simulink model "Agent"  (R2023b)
settings: Solver=ode3  StartTime=0.0  StopTime=t_end  FixedStep=dt8dof  RelTol=1e-3
PreLoadFcn:
  | define_swarm_buses(3, 1000);
model workspace (MAT data in the model file):
  dt8dof = 0.002
  dtastar = 0.1
  dtcontrol = 0.03
  id = 1
  phi_road0 = 0
  psi0 = 0
  slope_x_body0 = 0
  slope_y_body0 = 0
  t_end = 70
  teta0 = 0
  tetapunto0 = 0
  theta_road0 = 0
  velstart = 5
  wr0_FL = 3.15
  wr0_FR = 3.15
  wr0_RL = 3.15
  wr0_RR = 3.15
  x0 = 0
  y0 = 0
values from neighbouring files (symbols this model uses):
  scenario = evalin('base', 'scenario')    [apply_map_event.m]    (also in obstacle_brake_from_base.m; swarm_planner_helper2.m)

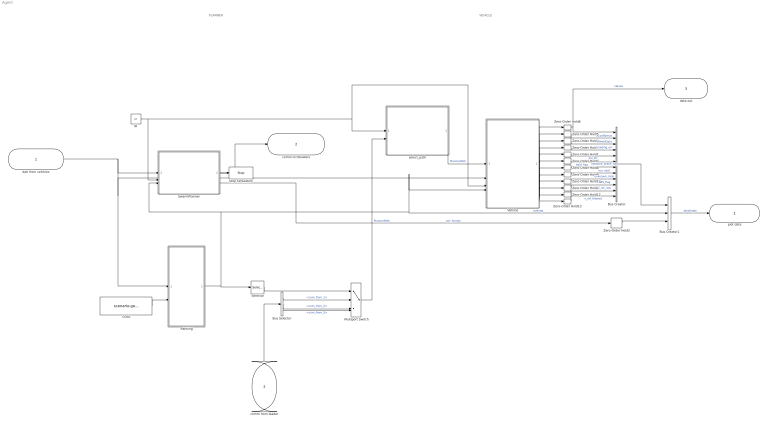
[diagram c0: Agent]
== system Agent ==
  note: PLANNER
  note: VEHICLE
  dati from vehicles : Inport  OutDataTypeStr=Bus: ValuesBus
  comm from leader : Inport  Port=2  OutDataTypeStr=Bus: PlannerOutBusGlobal  SampleTime=dtastar
  Bus Creator : BusCreator  Inputs=12  OutDataTypeStr=Bus: PlotVeicolo
  Bus Creator1 : BusCreator  Inputs=3  OutDataTypeStr=Bus: PlotSingle
  Bus Selector : BusSelector  OutputSignals=com_from_1,com_from_2,com_from_3
  GOAL : Constant  Value=scenario.goal
  ID : Constant  Value=id
  Multiport Switch : MultiPortSwitch
  Ranking : MATLAB Function  TreatAsAtomicUnit=on
  Selector : Selector  InputPortWidth=3  IndexOptions=Index vector (dialog)  Indices=[1]  OutputSizes=1
  Stop Simulation : Stop
  SwarmPlanner : MATLAB Function  TreatAsAtomicUnit=on
  Vehicle : ModelReference  ModelNameDialog=vehicle  UsingDefaultArgumentValue=0,0,0,0,0,0,0,0,0,0,0,0,0,0  SimulationMode=Normal  ModelReferenceVersion=1.119
  Zero-Order Hold{1..13} (13 alike) : ZeroOrderHold  SampleTime=dtastar
  select_path : MATLAB Function  TreatAsAtomicUnit=on
  plot data : Outport  OutDataTypeStr=Bus: PlotSingle  SampleTime=dtastar
  comm to followers : Outport  Port=2  OutDataTypeStr=Bus: PlannerOutBusSingle
  data out : Outport  Port=3  OutDataTypeStr=Bus: VehicleState
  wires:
  comm from leader/1 -> Bus Selector/1
  SwarmPlanner/1(PlannerOutBusSingle) -> comm to followers/1
  Bus Creator1/1 -> plot data/1  "plotsingle"
  ID/1 -> Vehicle/3, select_path/1(id), SwarmPlanner/2(id)
  Ranking/1(ranking) -> Selector/1, SwarmPlanner/3(ranking), Vehicle/4, Bus Creator1/2  "ranking"
  GOAL/1 -> Ranking/2(goal)
  Vehicle/2 -> Zero-Order Hold5/1
  Multiport Switch/1 -> select_path/2(Bus)  "PlannerPath"
  dati from vehicles/1 -> Ranking/1(ValuesBus), Vehicle/2, SwarmPlanner/1(ValuesBus)
  Vehicle/1 -> Zero-Order Hold6/1
  Bus Selector/1 -> Multiport Switch/2  "<com_from_1>"
  Bus Selector/2 -> Multiport Switch/3  "<com_from_2>"
  Bus Selector/3 -> Multiport Switch/4  "<com_from_3>"
  select_path/1(my_planner_data) -> Vehicle/1  "PlannerPath"
  SwarmPlanner/3(pct_known) -> Zero-Order Hold2/1  "pct_known"
  Bus Creator/1 -> Bus Creator1/1
  Vehicle/3 -> Zero-Order Hold4/1
  SwarmPlanner/2(goal_flag) -> Stop Simulation/1
  Zero-Order Hold2/1 -> Bus Creator1/3
  Selector/1 -> Multiport Switch/1
  Vehicle/5 -> Zero-Order Hold1/1
  Vehicle/4 -> Zero-Order Hold3/1
  Zero-Order Hold1/1 -> Bus Creator/5  "psi_err"
  Zero-Order Hold3/1 -> Bus Creator/4  "heading_err"
  Zero-Order Hold4/1 -> Bus Creator/3  "WheelData"
  Zero-Order Hold5/1 -> Bus Creator/2  "AccelSterzo"
  Zero-Order Hold6/1 -> Bus Creator/1, data out/1  "values"
  Zero-Order Hold7/1 -> Bus Creator/6  "obstacle_brake_flag"
  Vehicle/6 -> Zero-Order Hold7/1
  Zero-Order Hold8/1 -> Bus Creator/7  "hold_flag"
  Vehicle/7 -> Zero-Order Hold8/1
  Vehicle/8 -> Zero-Order Hold9/1
  Vehicle/12 -> Zero-Order Hold13/1
  Vehicle/11 -> Zero-Order Hold12/1
  Vehicle/10 -> Zero-Order Hold11/1
  Vehicle/9 -> Zero-Order Hold10/1
  Zero-Order Hold9/1 -> Bus Creator/8  "mu_next"
  Zero-Order Hold10/1 -> Bus Creator/9  "unknown_ratio"
  Zero-Order Hold11/1 -> Bus Creator/10  "ABS_flag"
  Zero-Order Hold12/1 -> Bus Creator/11  "v_ref_raw"
  Zero-Order Hold13/1 -> Bus Creator/12  "v_ref_filtered"
  ? -> ?

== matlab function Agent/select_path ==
function my_planner_data = select_my_path(id, Bus)
%SELECT_MY_PATH Estrae il PlannerPath del veicolo corrente.
%#codegen

my_planner_data = Bus.id1;

switch int32(id)
    case 1
        my_planner_data = Bus.id1;

    case 2
        my_planner_data = Bus.id2;

    case 3
        my_planner_data = Bus.id3;

    otherwise
        my_planner_data = Bus.id1;
end

end

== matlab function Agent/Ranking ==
function ranking = classifica(ValuesBus, goal)
%CLASSIFICA Ranking decentralizzato pesato:
% 70% distanza dal goal + 30% ETA radiale al goal, con isteresi.
%
% Score basso = veicolo migliore.
%
%#codegen

%% Parametri
N_VEH = 3;

W_DIST = 0.70;
W_ETA  = 0.30;

HYST_FRAC = 0.20;

% Velocita' radiale minima utile verso il goal.
% Sotto questa soglia considero l'ETA non affidabile.
V_RAD_EPS = 0.20;     % [m/s]

% Valore normalizzato assegnato a veicoli che non stanno andando verso il goal.
% 2.0 = penalita' moderata, non infinita.
% Se vuoi punire di piu' chi va nella direzione sbagliata, metti 3.0.
ETA_BAD_NORM = 2.0;

DIST_EPS = 1e-6;
ETA_EPS  = 1e-6;

%% Allocazione statica
ids = zeros(N_VEH, 1);

xs  = zeros(N_VEH, 1);
ys  = zeros(N_VEH, 1);
ps  = zeros(N_VEH, 1);
vs  = zeros(N_VEH, 1);

dist_arr = zeros(N_VEH, 1);
eta_arr  = zeros(N_VEH, 1);
eta_valid = false(N_VEH, 1);

scores = zeros(N_VEH, 1);

%% Raccolta stati statica dal bus

ids(1) = 1;
xs(1)  = ValuesBus.id1.x;
ys(1)  = ValuesBus.id1.y;
ps(1)  = ValuesBus.id1.psi;
vs(1)  = ValuesBus.id1.vel_totale;

ids(2) = 2;
xs(2)  = ValuesBus.id2.x;
ys(2)  = ValuesBus.id2.y;
ps(2)  = ValuesBus.id2.psi;
vs(2)  = ValuesBus.id2.vel_totale;

ids(3) = 3;
xs(3)  = ValuesBus.id3.x;
ys(3)  = ValuesBus.id3.y;
ps(3)  = ValuesBus.id3.psi;
vs(3)  = ValuesBus.id3.vel_totale;

%% Goal
gx = goal(1);
gy = goal(2);

%% Prima passata: calcolo distanze ed ETA radiali
for k = 1:N_VEH

    dx = gx - xs(k);
    dy = gy - ys(k);

    d = sqrt(dx*dx + dy*dy);
    dist_arr(k) = d;

    if d < 1e-3
        eta_arr(k) = 0.0;
        eta_valid(k) = true;
    else
        ux = dx / d;
        uy = dy / d;

        vx = vs(k) * cos(ps(k));
        vy = vs(k) * sin(ps(k));

        % Velocita' proiettata lungo la direzione veicolo -> goal
        v_rad = vx*ux + vy*uy;

        if v_rad > V_RAD_EPS
            eta_arr(k) = d / v_rad;
            eta_valid(k) = true;
        else
            % Veicolo fermo, laterale o che si sta allontanando dal goal.
            eta_arr(k) = 0.0;
            eta_valid(k) = false;
        end
    end
end

%% Normalizzazione distanza
d_ref = max(dist_arr);

if d_ref < DIST_EPS
    d_ref = 1.0;
end

%% Normalizzazione ETA solo sui veicoli validi
eta_ref = 0.0;

for k = 1:N_VEH
    if eta_valid(k)
        if eta_arr(k) > eta_ref
            eta_ref = eta_arr(k);
        end
    end
end

if eta_ref < ETA_EPS
    eta_ref = 1.0;
end

%% Score finale normalizzato
for k = 1:N_VEH

    d_norm = dist_arr(k) / d_ref;

    if eta_valid(k)
        eta_norm = eta_arr(k) / eta_ref;

        % Saturazione: il termine ETA non deve distruggere il peso 70/30.
        if eta_norm > ETA_BAD_NORM
            eta_norm = ETA_BAD_NORM;
        end
    else
        eta_norm = ETA_BAD_NORM;
    end

    scores(k) = W_DIST * d_norm + W_ETA * eta_norm;
end

%% Ordina e applica isteresi
[sorted_sc, idx_sorted] = sort(scores);
new_ranking = ids(idx_sorted);

persistent prev_ranking

if isempty(prev_ranking)
    prev_ranking = new_ranking;
    ranking = new_ranking;
    return;
end

if isequal(new_ranking, prev_ranking)

    ranking = new_ranking;

else

    best_score   = sorted_sc(1);
    second_score = sorted_sc(2);

    % Se il vantaggio del nuovo primo e' piccolo, mantieni il ranking precedente.
    if abs(second_score - best_score) < HYST_FRAC * max(second_score, 1e-6)
        ranking = prev_ranking;
    else
        ranking = new_ranking;
        prev_ranking = new_ranking;
    end

end

end

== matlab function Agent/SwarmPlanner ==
function [PlannerOutBusSingle, goal_flag, pct_known] = ...
    SwarmPlanner(ValuesBus, id, ranking)
%SWARMPLANNER Wrapper Simulink per architettura decentralizzata.
%
% ranking = [id_primo; id_secondo; id_terzo]
%
% path_x_1 = path per il primo classificato
% path_x_2 = path per il secondo classificato
% path_x_3 = path per il terzo classificato
%
% L'output finale viene rimappato su:
% PlannerOutBusSingle.id1 / id2 / id3
%
%#codegen

coder.extrinsic('swarm_planner_rank_to_id');

L        = 1000; 
N_REPLAN = 2;

%% Default scalari
goal_flag = 0.0;
pct_known = 0.0;

%% Default bus output: necessario SEMPRE, anche se non sono leader
z = zeros(L,1);

PlannerOutBusSingle.id1.to_path_tracker.path_x = z;
PlannerOutBusSingle.id1.to_path_tracker.path_y = z;
PlannerOutBusSingle.id1.to_path_tracker.n      = 0.0;
PlannerOutBusSingle.id1.to_speed_governor.mu_next       = 1; %metto mu alta, sarà soltanto la prima del segnale disceto,
% altrimenti lo speederefence governor la prima mu che legge è 0 e porta vref=0
PlannerOutBusSingle.id1.to_speed_governor.unknown_ratio = 0.0;

PlannerOutBusSingle.id2.to_path_tracker.path_x = z;
PlannerOutBusSingle.id2.to_path_tracker.path_y = z;
PlannerOutBusSingle.id2.to_path_tracker.n      = 0.0;
PlannerOutBusSingle.id2.to_speed_governor.mu_next       = 1;
PlannerOutBusSingle.id2.to_speed_governor.unknown_ratio = 0.0;

PlannerOutBusSingle.id3.to_path_tracker.path_x = z;
PlannerOutBusSingle.id3.to_path_tracker.path_y = z;
PlannerOutBusSingle.id3.to_path_tracker.n      = 0.0;
PlannerOutBusSingle.id3.to_speed_governor.mu_next       = 1;
PlannerOutBusSingle.id3.to_speed_governor.unknown_ratio = 0.0;

%% Se NON sono primo in classifica, esco con bus zero
if int32(ranking(1)) ~= int32(id)
    return;
end

%% Lettura stati con campi STATICI
x_id1   = ValuesBus.id1.x;
y_id1   = ValuesBus.id1.y;
psi_id1 = ValuesBus.id1.psi;

x_id2   = ValuesBus.id2.x;
y_id2   = ValuesBus.id2.y;
psi_id2 = ValuesBus.id2.psi;

x_id3   = ValuesBus.id3.x;
y_id3   = ValuesBus.id3.y;
psi_id3 = ValuesBus.id3.psi;

%% Buffer numerico già rimappato in ordine id1/id2/id3
buf = zeros(6*L + 11, 1);

buf = swarm_planner_rank_to_id( ...
    x_id1, y_id1, psi_id1, ...
    x_id2, y_id2, psi_id2, ...
    x_id3, y_id3, psi_id3, ...
    ranking, L, N_REPLAN);

%% Unpack: ora i dati sono in ordine ID fisso, NON in ordine classifica
path_x_id1 = buf(1:L);
path_y_id1 = buf(L+1:2*L);
n_id1      = buf(2*L+1);

path_x_id2 = buf(2*L+2:3*L+1);
path_y_id2 = buf(3*L+2:4*L+1);
n_id2      = buf(4*L+2);

path_x_id3 = buf(4*L+3:5*L+2);
path_y_id3 = buf(5*L+3:6*L+2);
n_id3      = buf(6*L+3);

goal_flag = buf(6*L+4);
pct_known = buf(6*L+5);

mu_id1 = buf(6*L+6);
mu_id2 = buf(6*L+7);
mu_id3 = buf(6*L+8);

unk_id1 = buf(6*L+9);
unk_id2 = buf(6*L+10);
unk_id3 = buf(6*L+11);

%% Assemblaggio bus con campi STATICI
PlannerOutBusSingle.id1.to_path_tracker.path_x = path_x_id1;
PlannerOutBusSingle.id1.to_path_tracker.path_y = path_y_id1;
PlannerOutBusSingle.id1.to_path_tracker.n      = n_id1;
PlannerOutBusSingle.id1.to_speed_governor.mu_next       = mu_id1;
PlannerOutBusSingle.id1.to_speed_governor.unknown_ratio = unk_id1;

PlannerOutBusSingle.id2.to_path_tracker.path_x = path_x_id2;
PlannerOutBusSingle.id2.to_path_tracker.path_y = path_y_id2;
PlannerOutBusSingle.id2.to_path_tracker.n      = n_id2;
PlannerOutBusSingle.id2.to_speed_governor.mu_next       = mu_id2;
PlannerOutBusSingle.id2.to_speed_governor.unknown_ratio = unk_id2;

PlannerOutBusSingle.id3.to_path_tracker.path_x = path_x_id3;
PlannerOutBusSingle.id3.to_path_tracker.path_y = path_y_id3;
PlannerOutBusSingle.id3.to_path_tracker.n      = n_id3;
PlannerOutBusSingle.id3.to_speed_governor.mu_next       = mu_id3;
PlannerOutBusSingle.id3.to_speed_governor.unknown_ratio = unk_id3;

end
